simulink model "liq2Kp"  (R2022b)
settings: Solver=ode45  StartTime=0.0  StopTime=60*10  FixedStep=1  RelTol=1e-6  EnableMultiTasking=on
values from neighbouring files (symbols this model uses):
  a = k12/(2*Ar*sqrt(h1b-h2b))    [para2Kp.m]    (also in nyqlog.m = log(spiralfactor)*2/pi)
  Ar = 6*25.4    (= 152.4)    [para2Kp.m]
  b = k2/(2*Ar*sqrt(h2b))    [para2Kp.m]
  h2b = (qb/k2)^2    (= 5.00000710049)    [para2Kp.m]
  k1 = 0    [para2Kp.m]
  k12 = 38    [para2Kp.m]
  k2 = 11.5    [para2Kp.m]
  Kp = 10    [para2Kp.m]
  qb = 25.7148    [para2Kp.m]
  qmax = 90    [para2Kp.m]
  qmin = -85    [para2Kp.m]
libraries: simulink x1

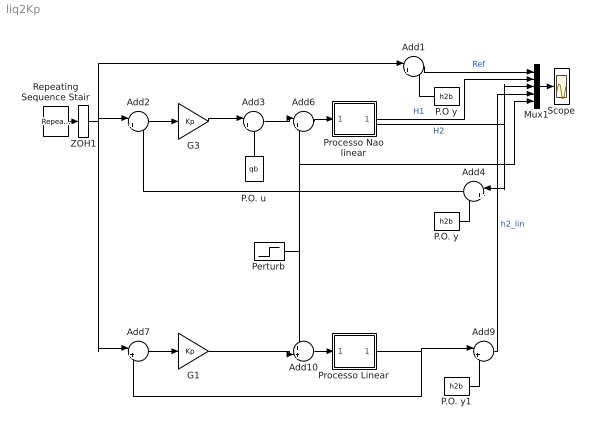
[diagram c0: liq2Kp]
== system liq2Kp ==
  Add{1,3,6,9} (4 alike) : Sum  Inputs=|++
  Add10 : Sum  Inputs=++|
  Add2 : Sum  Inputs=|+-
  Add4 : Sum  Inputs=|+-
  Add7 : Sum  Inputs=|+-
  G1 : Gain  Gain=Kp
  G3 : Gain  Gain=Kp
  Mux1 : Mux  Inputs=5
  P.O y : Constant  Value=h2b
  P.O. u : Constant  Value=qb
  P.O. y : Constant  Value=h2b
  P.O. y1 : Constant  Value=h2b
  Perturb : Step  Time=500  After=10  SampleTime=0
  Processo Nao linear : Subsystem
  Processo Linear : Subsystem
  Repeating Sequence Stair : simulink/Sources/Repeating Sequence Stair  OutValues=[2 5 12 5 2].'-h2b  tsamp=100  OutMin=[]  OutMax=[]  OutDataTypeStr=double  OutputDataTypeScalingMode=double  OutDataType=fixdt(0,8)  ConRadixGroup=Best Precision: Vector-wise  OutScaling=2^-12
  Scope : Scope
  ZOH1 : ZeroOrderHold
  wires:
  Mux1/1 -> Scope/1
  Add2/1 -> G3/1
  Processo Nao linear/2(H2) -> Mux1/3, Add4/1  "H2"
  ZOH1/1 -> Add7/1, Add2/1, Add1/1
  P.O. u/1 -> Add3/2
  P.O y/1 -> Add1/2
  Add1/1 -> Mux1/1  "Ref"
  P.O. y/1 -> Add4/2
  Processo Nao linear/1(H1) -> Mux1/2  "H1"
  Repeating Sequence Stair/1 -> ZOH1/1
  Perturb/1 -> Add10/1, Mux1/5, Add6/2
  Add6/1 -> Processo Nao linear/1(u)
  G3/1 -> Add3/1
  Add4/1 -> Add2/2
  Add7/1 -> G1/1
  P.O. y1/1 -> Add9/2
  Add10/1 -> Processo Linear/1(ul)
  Processo Linear/1(h2) -> Add9/1, Add7/2
  G1/1 -> Add10/2
  Add9/1 -> Mux1/4  "h2_lin"
  Add3/1 -> Add6/1

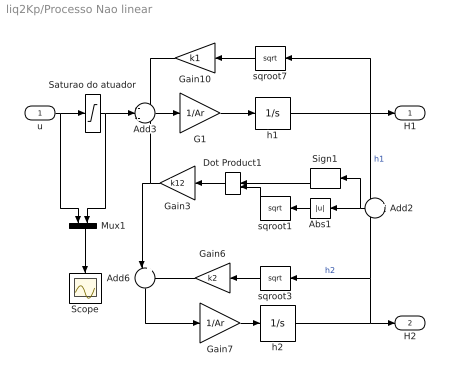
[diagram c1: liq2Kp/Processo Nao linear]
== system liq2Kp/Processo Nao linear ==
  u : Inport
  Abs1 : Abs
  Add2 : Sum  Inputs=+-
  Add3 : Sum  Inputs=-+-
  Add6 : Sum  Inputs=|+-
  Dot Product1 : DotProduct
  G1 : Gain  Gain=1/Ar
  Gain10 : Gain  Gain=k1
  Gain3 : Gain  Gain=k12
  Gain6 : Gain  Gain=k2
  Gain7 : Gain  Gain=1/Ar
  Mux1 : Mux  Inputs=2
  Saturao do atuador : Saturate  UpperLimit=qmax  LowerLimit=qmin
  Scope : Scope
  Sign1 : Signum
  h1 : Integrator  LimitOutput=on  UpperSaturationLimit=16.5  LowerSaturationLimit=0
  h2 : Integrator  LimitOutput=on  UpperSaturationLimit=16.5  LowerSaturationLimit=0
  sqroot1 : Math  Operator=sqrt  SignedPower=on
  sqroot3 : Math  Operator=sqrt  SignedPower=on
  sqroot7 : Math  Operator=sqrt  SignedPower=on
  H1 : Outport  VectorParamsAs1DForOutWhenUnconnected=off
  H2 : Outport  Port=2  VectorParamsAs1DForOutWhenUnconnected=off
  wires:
  h1/1 -> Add2/1, H1/1, sqroot7/1  "h1"
  h2/1 -> Add2/2, sqroot3/1, H2/1  "h2"
  Saturao do atuador/1 -> Add3/2, Mux1/2
  Add6/1 -> Gain7/1
  Gain10/1 -> Add3/1
  sqroot7/1 -> Gain10/1
  Gain6/1 -> Add6/2
  Gain7/1 -> h2/1
  sqroot3/1 -> Gain6/1
  G1/1 -> h1/1
  Gain3/1 -> Add6/1, Add3/3
  Add3/1 -> G1/1
  Dot Product1/1 -> Gain3/1
  sqroot1/1 -> Dot Product1/2
  Sign1/1 -> Dot Product1/1
  Abs1/1 -> sqroot1/1
  Add2/1 -> Abs1/1, Sign1/1
  u/1 -> Saturao do atuador/1, Mux1/1
  Mux1/1 -> Scope/1

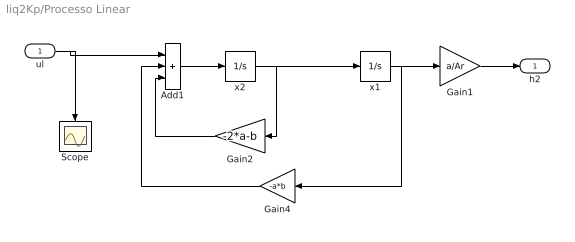
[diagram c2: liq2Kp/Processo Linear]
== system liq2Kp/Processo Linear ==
  ul : Inport
  Add1 : Sum  Inputs=+++
  Gain1 : Gain  Gain=a/Ar
  Gain2 : Gain  Gain=-2*a-b
  Gain4 : Gain  Gain=-a*b
  Scope : Scope
  x1 : Integrator
  x2 : Integrator
  h2 : Outport  VectorParamsAs1DForOutWhenUnconnected=off
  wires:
  ul/1 -> Scope/1, Add1/1
  x1/1 -> Gain4/1, Gain1/1
  x2/1 -> Gain2/1, x1/1
  Gain1/1 -> h2/1
  Add1/1 -> x2/1
  Gain2/1 -> Add1/3
  Gain4/1 -> Add1/2
